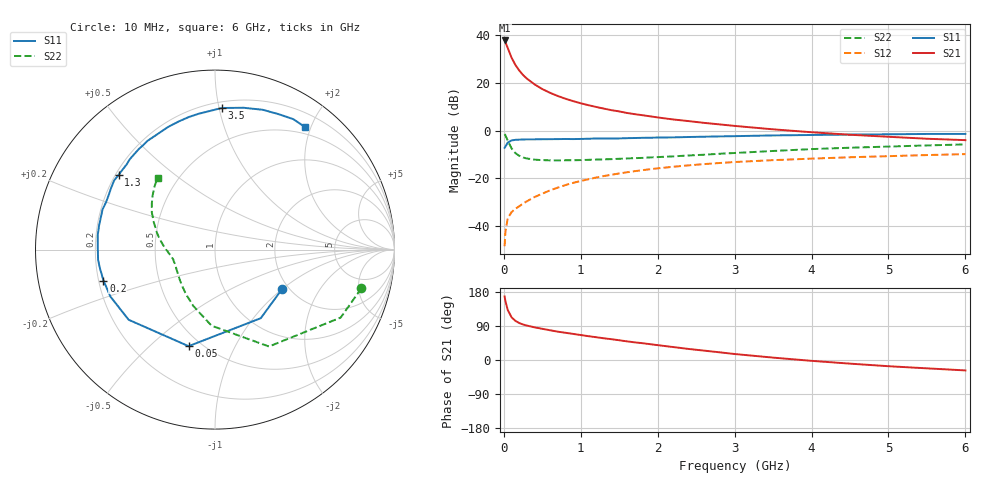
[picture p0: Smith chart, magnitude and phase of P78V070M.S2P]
! SIEMENS Small Signal Semiconductors
! BFP196
! Si NPN RF Bipolar Junction Transistor in SOT143
! VCE = 8 V  IC = 70 mA
! Common Emitter S-Parameters:  May  1996
# GHz  S  MA  R  50
!  f  S11  S21  S12  S22
! GHz  MAG  ANG  MAG  ANG  MAG  ANG  MAG  ANG
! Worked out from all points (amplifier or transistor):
!   36 points, 10 MHz to 6 GHz, reference 50 ohm
!   highest |S21| = 37.7 dB at 10 MHz (marker M1)
!   |S21| within 3 dB of that: start of sweep to 48.9 MHz
!   unconditionally stable (mu >= 1): 450.1 MHz to 4.622 GHz
!   at 250 MHz: K = 0.84, MSG = 26.9 dB, |S12| = -30.6 dB
!   at 1.4 GHz: K = 1.09, MAG = 11.7 dB, |S12| = -18.5 dB
!   at 6 GHz: K = 0.98, MSG = 2.9 dB, |S12| = -9.9 dB
!   S11 on the Smith chart (normalised r, x): 10 MHz: 1.86, -1.00; 50 MHz: 0.43, -0.67; 200 MHz: 0.22, -0.13; 1.3 GHz: 0.21, +0.33; 3.5 GHz: 0.24, +1.02; 6 GHz: 0.40, +1.92
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0.01  0.434 -30.1  76.71 167.7  0.0038 78.7  0.8438 -14.8
0.02  0.4594 -56.3  71.14 156.1  0.0074 71.5  0.7961 -28.4
0.05  0.5578 -105.3  53.75 132.4  0.0145 56.2  0.6179 -60.9
0.1  0.6199 -140.9  33.53 112.8  0.0196 48.3  0.4243 -92.6
0.15  0.6388 -155.8  23.59 103.3  0.023 48.7  0.337 -110.9
0.2  0.6448 -164.5  18.09 97.6  0.026 50.9  0.296 -123.2
0.25  0.6493 -170.6  14.52 93.6  0.0296 54.1  0.2723 -132.4
0.3  0.6539 -174.9  12.19 90.8  0.0331 56.7  0.2599 -138.6
0.4  0.6539 177.9  9.226 86.2  0.0406 59.6  0.2459 -147.9
0.5  0.6584 173.1  7.371 82.3  0.0478 61.3  0.2399 -154.0
0.6  0.6596 168.2  6.163 78.5  0.0559 61.8  0.2376 -158.2
0.7  0.661 164.0  5.291 74.8  0.0638 62.5  0.2372 -161.3
0.9  0.662 156.6  4.124 68.9  0.0802 61.2  0.2386 -166.2
1.1  0.6732 149.3  3.389 62.9  0.0956 59.6  0.2437 -169.4
1.3  0.679 142.3  2.874 57.3  0.1115 57.3  0.2491 -172.4
1.7  0.6968 130.1  2.2 46.6  0.1409 51.9  0.264 -177.9
2.2  0.7186 116.5  1.706 34.2  0.1743 44.6  0.2877 175.6
2.8  0.7531 101.1  1.346 20.4  0.2087 35.7  0.326 166.3
3.5  0.79 87.2  1.059 6.3  0.2399 25.8  0.3733 156.0
4.5  0.8233 71.1  0.816 -9.6  0.2757 14.0  0.4366 143.7
5.5  0.8477 59.0  0.673 -22.0  0.3064 3.4  0.4878 133.6
6  0.8473 53.5  0.629 -27.5  0.3211 -2.2  0.5122 128.7
